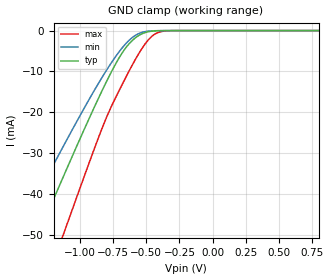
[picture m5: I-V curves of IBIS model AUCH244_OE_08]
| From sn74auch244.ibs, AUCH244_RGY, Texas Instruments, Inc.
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[Model]   AUCH244_OE_08
Model_type  Input
Vinl=0.28
Vinh=0.52
| variable   typ   min   max
C_comp   2.61pF   2.27pF   2.92pF
[Temperature Range]   40   100   -40
| Ambient temperature   25   85   -40
[Voltage range]   0.8   0.8   0.8
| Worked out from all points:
|   GND clamp passes 1 mA (typ) near -0.55 V on its own axis
[GND Clamp]
| AUCH244_OE_08
|   Voltage   I(typ)   I(min)   I(max)
-3.6V     -226.6mA   -190.3mA   -271.8mA
-1.485V   -63.01mA   -50.7mA    -82.58mA
-1.445V   -59.95mA   -48.16mA   -78.96mA
-1.305V   -49.28mA   -39.36mA   -66.26mA
-1.135V   -36.48mA   -28.9mA    -50.82mA
-1.1V     -33.88mA   -26.79mA   -47.64mA
-840mV    -15.17mA   -11.81mA   -24.5mA
-695mV    -6.152mA   -4.773mA   -14.06mA
-580mV    -1.726mA   -1.13mA    -6.949mA
-450mV    -123.7uA   -59.61uA   -1.212mA
-315mV    -2.431uA   -1.534uA   -21.15uA
800mV     96.17pA    180.2pA    76.88pA
